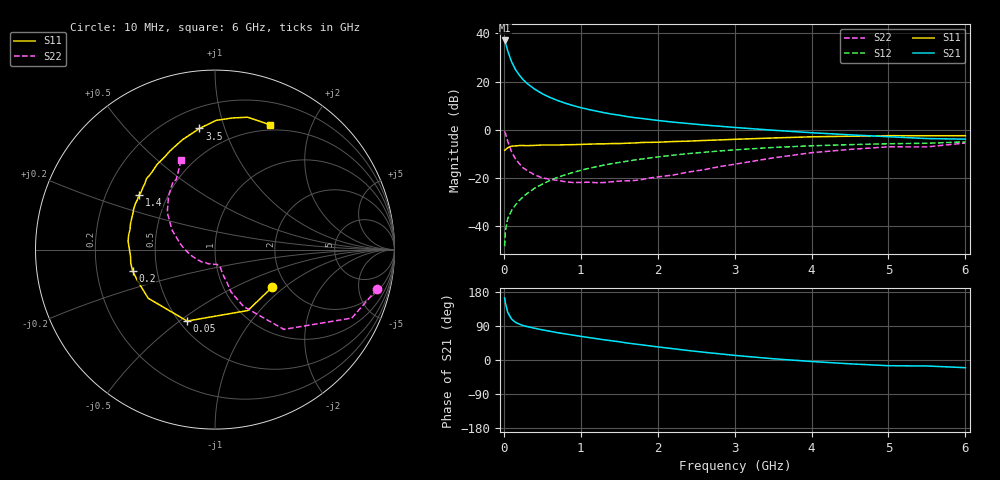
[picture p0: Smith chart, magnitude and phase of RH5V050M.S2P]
! SIEMENS Small Signal Semiconductors
! BFR106
! Si NPN RF Bipolar Junction Transistor in SOT23
! VCE = 5 V  IC = 50 mA
! Common Emitter S-Parameters:  August  1996
# GHz  S  MA  R  50
!  f  S11  S21  S12  S22
! GHz  MAG  ANG  MAG  ANG  MAG  ANG  MAG  ANG
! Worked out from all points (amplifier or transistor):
!   36 points, 10 MHz to 6 GHz, reference 50 ohm
!   highest |S21| = 37.1 dB at 10 MHz (marker M1)
!   |S21| within 3 dB of that: start of sweep to 38.88 MHz
!   unconditionally stable (mu >= 1): 248.3 MHz to 2.232 GHz
!   at 250 MHz: K = 1.00, MAG = 24.0 dB, |S12| = -27.7 dB
!   at 1.4 GHz: K = 1.06, MAG = 8.8 dB, |S12| = -14.0 dB
!   at 6 GHz: K = 0.99, MSG = 0.6 dB, |S12| = -5.0 dB
!   S11 on the Smith chart (normalised r, x): 10 MHz: 1.69, -0.82; 50 MHz: 0.55, -0.53; 200 MHz: 0.36, -0.11; 1.4 GHz: 0.34, +0.29; 3.5 GHz: 0.33, +0.83; 6 GHz: 0.44, +1.44
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0.01  0.3815 -33.1  71.37 163.8  0.0039 80.6  0.9289 -13.8
0.02  0.3856 -61.7  64.62 150.9  0.008 69.3  0.8522 -26.6
0.05  0.4272 -111.3  43.72 125.7  0.0145 60.6  0.5872 -49.2
0.1  0.4604 -143.9  25.93 108.2  0.0213 61.4  0.3539 -63.4
0.15  0.4655 -158.2  17.93 99.6  0.0277 64.2  0.2534 -69.2
0.2  0.4744 -165.6  13.72 94.8  0.0344 67.4  0.2001 -69.9
0.25  0.4751 -171.1  11 91.0  0.0411 68.9  0.164 -71.4
0.3  0.4721 -175.0  9.24 88.3  0.0479 70.5  0.145 -72.3
0.4  0.4775 179.3  6.996 83.8  0.0619 71.5  0.1172 -73.1
0.5  0.4865 174.6  5.613 79.6  0.0753 71.7  0.1015 -73.4
0.6  0.4879 170.6  4.701 75.8  0.0901 71.3  0.0949 -75.4
0.7  0.4867 166.7  4.064 72.0  0.1041 70.9  0.0899 -78.8
0.9  0.4949 160.2  3.191 65.6  0.1318 68.7  0.0813 -84.0
1.1  0.5066 153.5  2.656 59.4  0.1592 66.3  0.0825 -94.2
1.4  0.5212 144.4  2.128 50.8  0.1992 62.3  0.0842 -108.5
1.7  0.5368 136.7  1.796 42.3  0.2376 58.0  0.0897 -126.5
2.2  0.574 124.2  1.45 29.8  0.2994 50.6  0.1162 -153.4
2.8  0.6201 110.4  1.194 16.4  0.3654 41.5  0.1735 177.8
3.5  0.6805 97.3  0.985 3.3  0.4328 31.0  0.2632 155.5
4.5  0.7397 82.5  0.791 -10.1  0.4948 16.4  0.3948 131.0
5.5  0.7574 70.4  0.662 -15.8  0.5294 6.7  0.4446 119.1
6  0.7588 66.2  0.644 -20.3  0.5646 -0.5  0.5355 110.5
